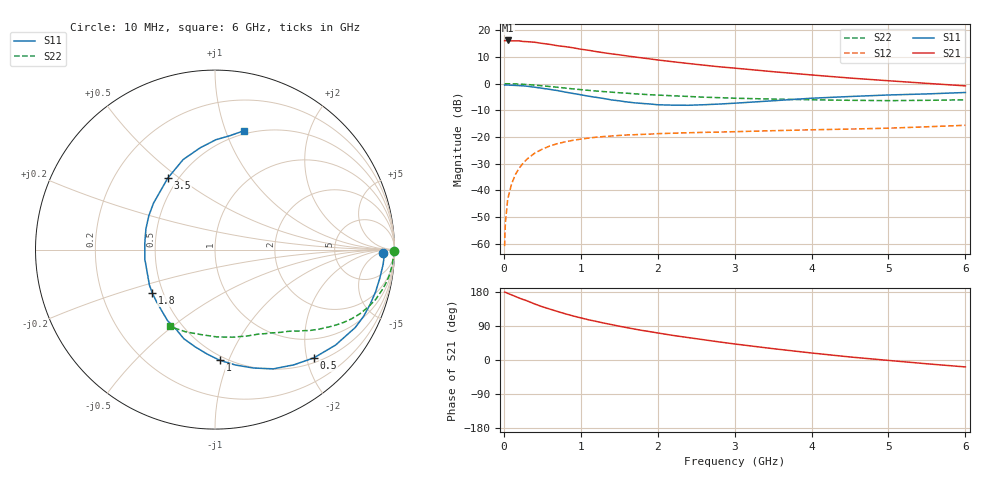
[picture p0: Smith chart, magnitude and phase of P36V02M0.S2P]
! SIEMENS Small Signal Semiconductors
! BFP181
! Si NPN RF Bipolar Junction Transistor in SOT143
! VCE = 6 V  IC = 2 mA
! Common Emitter S-Parameters:  March  1996
# GHz  S  MA  R  50
!  f  S11  S21  S12  S22
! GHz  MAG  ANG  MAG  ANG  MAG  ANG  MAG  ANG
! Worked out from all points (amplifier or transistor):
!   36 points, 10 MHz to 6 GHz, reference 50 ohm
!   highest |S21| = 16.2 dB at 50 MHz (marker M1)
!   |S21| within 3 dB of that: start of sweep to 948 MHz
!   unconditionally stable (mu >= 1): 2.544 GHz to end of sweep
!   at 250 MHz: K = 0.12, MSG = 22.8 dB, |S12| = -29.8 dB
!   at 1.4 GHz: K = 0.63, MSG = 15.4 dB, |S12| = -19.6 dB
!   at 6 GHz: K = 1.14, MAG = 5.1 dB, |S12| = -15.6 dB
!   lowest NFmin = 1.35 dB at 450 MHz
!   S11 on the Smith chart (normalised r, x): 10 MHz: 29, -9; 500 MHz: 0.59, -2.14; 1 GHz: 0.47, -0.93; 1.8 GHz: 0.44, -0.26; 3.5 GHz: 0.44, +0.45; 6 GHz: 0.47, +1.16
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0.01  0.9389 -1.2  6.375 179.2  0.0009 77.0  0.9965 -0.4
0.02  0.9433 -2.1  6.379 178.7  0.0024 84.6  0.9935 -0.9
0.05  0.9404 -5.0  6.434 175.9  0.0068 88.8  0.9939 -2.3
0.1  0.9319 -9.9  6.314 171.9  0.0131 83.2  0.9917 -4.5
0.2  0.9161 -19.7  6.316 163.5  0.0261 78.2  0.9796 -9.0
0.4  0.8567 -38.4  5.962 147.9  0.0496 66.8  0.9376 -17.2
0.5  0.8173 -47.5  5.667 140.6  0.0592 61.6  0.9097 -20.8
0.6  0.7781 -55.6  5.426 134.2  0.068 57.4  0.882 -24.0
0.7  0.7398 -63.9  5.116 127.9  0.0753 53.3  0.8529 -26.9
0.8  0.6934 -72.1  4.926 121.8  0.0812 49.2  0.8249 -29.4
0.9  0.6532 -79.9  4.689 116.3  0.0868 45.8  0.796 -31.8
1  0.6176 -87.5  4.414 111.2  0.0911 42.8  0.7705 -33.9
1.1  0.5822 -94.6  4.214 106.2  0.0954 40.3  0.7472 -35.8
1.3  0.526 -109.3  3.785 97.5  0.102 35.6  0.7083 -39.2
1.5  0.4761 -123.7  3.465 89.2  0.1068 31.9  0.6741 -42.0
1.8  0.4247 -145.4  3.028 78.0  0.1119 28.0  0.6315 -45.9
2.2  0.3945 -172.2  2.566 64.8  0.1177 23.7  0.5915 -51.1
2.8  0.414 153.0  2.067 47.7  0.1236 19.5  0.5454 -59.2
3.5  0.4771 123.5  1.672 29.9  0.1312 16.4  0.5134 -69.7
4.5  0.5731 98.3  1.271 8.0  0.1407 12.7  0.4865 -88.8
5.5  0.6409 82.4  1.011 -10.0  0.1553 11.0  0.4864 -109.6
6  0.6817 76.3  0.907 -18.3  0.1656 9.1  0.4968 -120.5
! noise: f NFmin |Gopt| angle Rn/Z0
0.45  1.35  0.6  17  0.4
0.9  1.45  0.5  36  0.4
1.8  1.8  0.31  80  0.37
